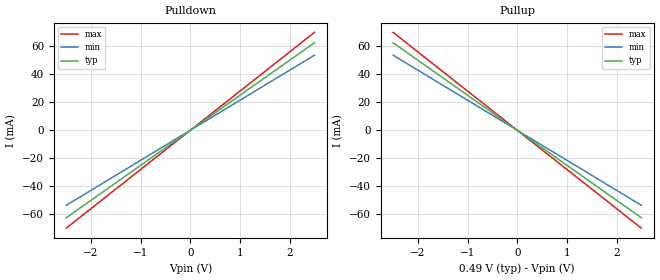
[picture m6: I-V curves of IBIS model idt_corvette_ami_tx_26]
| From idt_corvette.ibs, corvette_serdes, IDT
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|   model   idt_corvette_ami_tx_26
[Model] idt_corvette_ami_tx_26
Model_type Output
C_comp 400f 400f 400f
Cref = 0
[Model Spec]
Vmeas 0. 0. 0.
Vref 0. 0. 0.
[Temperature Range]  25 100 0
[Voltage Range] .49 .499 .419
[Algorithmic Model]
Executable Windows_VisualStudio5_32 idt_corvette_tx.dll   idt_corvette_tx.ami
Executable Windows_ver_64   idt_corvette_tx_64.dll   idt_corvette_tx.ami
Executable Linux_gcc4.1.2_32   idt_corvette_tx.linux.so   idt_corvette_tx.ami
Executable Linux_gcc3.2.3_64   idt_corvette_tx_64.linux.so idt_corvette_tx.ami
[End Algorithmic Model]
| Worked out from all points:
|   slope of the pulldown table from 0 to 0.073 V, typ, clamps not added: 40 ohm
|   slope of the pullup table from 0 to 0.073 V, typ, clamps not added: 40 ohm
[Pulldown]
-2.5V     -62.5mA    -53.62mA   -69.92mA
0V        0A         0A         0A
2.5V      62.5mA     53.62mA    69.92mA
[Pullup]
-2.5V     62.5mA     53.62mA    69.92mA
0V        0A         0A         0A
2.5V      -62.5mA    -53.62mA   -69.92mA
[Ramp]
dV/dt_r .163/22.4p .155/26.11p .147/20.022p
dV/dt_f .163/22.4p .155/26.11p .147/20.022p
